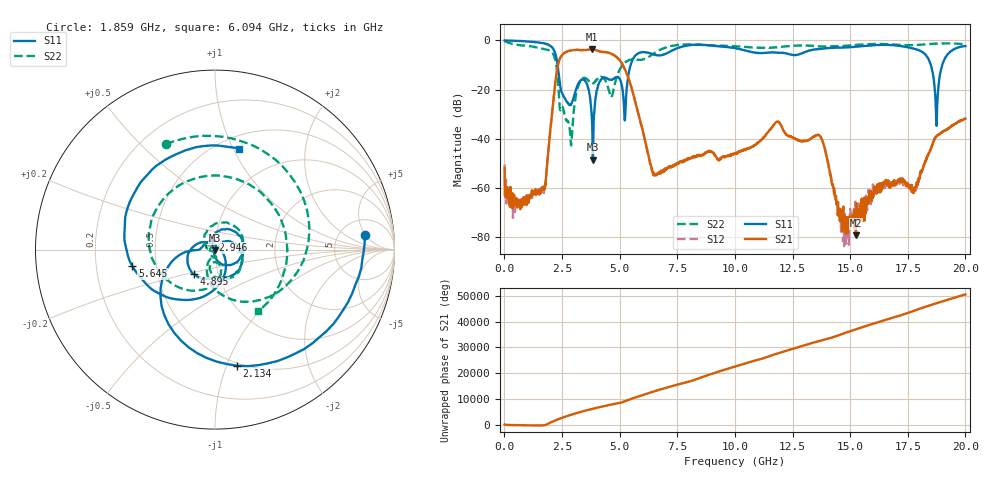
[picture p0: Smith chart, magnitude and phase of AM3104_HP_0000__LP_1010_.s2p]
!Created with skrf (http://scikit-rf.org).
# Hz S RI R 50.0
!freq ReS11 ImS11 ReS21 ImS21 ReS12 ImS12 ReS22 ImS22
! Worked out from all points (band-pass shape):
!   1601 points, 10 MHz to 20 GHz, reference 50 ohm
!   highest |S21| = -3.55 dB at 3.808 GHz (marker M1); lowest = -79.5 dB at 15.25 GHz (marker M2)
!   |S21| within 3 dB of the highest: 2.454 GHz to 4.842 GHz (2.388 GHz wide, 65.5 % of centre)
!   lowest |S11| = -48.6 dB at 3.833 GHz (marker M3), VSWR 1.01, Z = 49.8 - j0.326 ohm
!   |S11| at or under -10 dB: 2.306 GHz to 5.477 GHz (3.171 GHz wide, 81.5 % of centre); 18.5 GHz to 18.99 GHz (491.7 MHz wide, 2.62 % of centre)
!   |S22| runs from -42.8 to -0.2 dB; largest |S21 - S12| = 0.0047
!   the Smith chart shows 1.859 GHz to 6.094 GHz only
!   S11 on the Smith chart (normalised r, x): 1.859 GHz: 8.58, +4.80; 2.134 GHz: 0.48, -1.09; 2.946 GHz: 0.97, +0.10; 4.895 GHz: 0.76, -0.22; 5.645 GHz: 0.36, -0.09; 6.094 GHz: 0.63, +1.06
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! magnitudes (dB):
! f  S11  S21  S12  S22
! 10 MHz  0.0  -51.9  -50.6  -0.2
! 709.6 MHz  -0.2  -67.0  -66.1  -2.0
! 1.859 GHz  -1.5  -50.2  -50.0  -3.8
! 2.134 GHz  -3.6  -23.5  -23.5  -5.8
! 2.946 GHz  -25.0  -4.0  -4.0  -36.8
! 3.346 GHz  -15.9  -4.0  -4.0  -15.9
! 3.808 GHz  -34.4  -3.5  -3.5  -17.5
! 3.833 GHz  -48.6  -3.6  -3.6  -17.5
! 4.895 GHz  -14.9  -7.0  -7.0  -14.2
! 5.232 GHz  -32.3  -11.8  -11.8  -9.0
! 5.645 GHz  -6.6  -23.7  -23.7  -7.7
! 6.094 GHz  -4.8  -40.5  -40.5  -7.5
! 6.682 GHz  -6.1  -54.0  -54.0  -4.2
! 10.01 GHz  -3.1  -46.1  -46.1  -2.3
! 13.34 GHz  -3.8  -39.8  -39.8  -2.2
! 13.8 GHz  -3.3  -41.2  -41.1  -2.4
! 14.7 GHz  -2.9  -67.7  -75.5  -2.2
! 15.25 GHz  -2.5  -79.5  -70.8  -1.9
! 16.68 GHz  -1.8  -57.4  -58.6  -1.6
! 18.26 GHz  -5.7  -49.6  -49.5  -1.6
! 18.75 GHz  -34.8  -39.0  -39.0  -1.3
! 20 GHz  -2.3  -31.9  -31.9  -1.6
